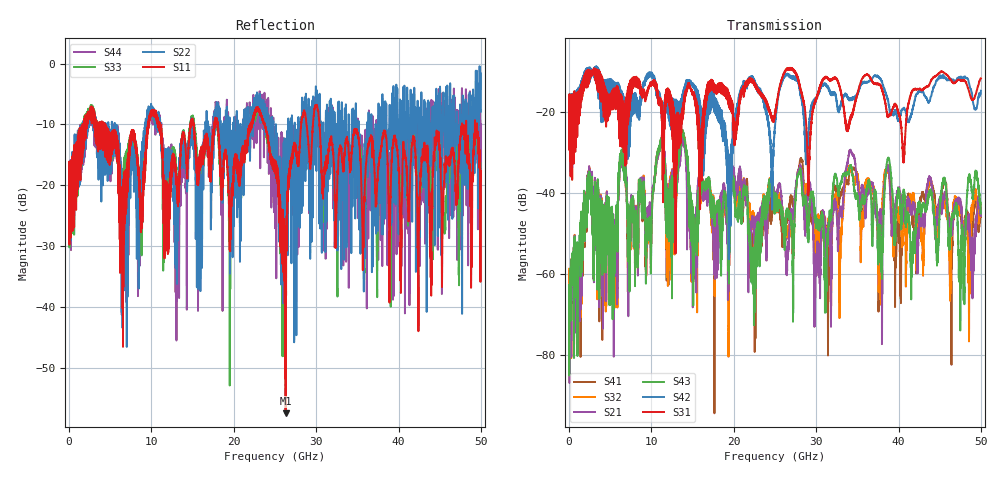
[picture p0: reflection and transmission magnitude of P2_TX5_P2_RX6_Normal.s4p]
!Keysight Technologies,N5225B,MY57041031,A.13.20.10
!Date: Friday, May 31, 2019 11:36:14
!Correction: S11(Full 4 Port(1,2,3,4))
!S12(Full 4 Port(1,2,3,4))
!S13(Full 4 Port(1,2,3,4))
!S14(Full 4 Port(1,2,3,4))
!S21(Full 4 Port(1,2,3,4))
!S22(Full 4 Port(1,2,3,4))
!S23(Full 4 Port(1,2,3,4))
!S24(Full 4 Port(1,2,3,4))
!S31(Full 4 Port(1,2,3,4))
!S32(Full 4 Port(1,2,3,4))
!S33(Full 4 Port(1,2,3,4))
!S34(Full 4 Port(1,2,3,4))
!S41(Full 4 Port(1,2,3,4))
!S42(Full 4 Port(1,2,3,4))
!S43(Full 4 Port(1,2,3,4))
!S44(Full 4 Port(1,2,3,4))
!S4P File: Measurements: <S11,S12,S13,S14>,
!<S21,S22,S23,S24>,
!<S31,S32,S33,S34>,
!<S41,S42,S43,S44>:
# Hz S  dB  R 50.0
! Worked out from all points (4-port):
!   5000 points, 10 MHz to 50 GHz, reference 50 ohm
!   strongest paths, dB at 10 MHz, 12.51 GHz, 25.01 GHz, 37.51 GHz, 50 GHz:
!     S31: -19.5, -17.7, -21.0, -13.1, -11.7
!     S42: -19.4, -16.8, -23.5, -11.2, -14.8
!     S43: -74.7, -40.7, -43.9, -52.8, -45.1
!     S21: -65.9, -37.4, -41.6, -51.0, -45.6
!     S32: -58.7, -37.5, -42.2, -56.1, -43.0
!     S41: -59.1, -39.3, -43.6, -54.7, -45.9
!   lowest |S11| = -57.5 dB at 26.29 GHz (marker M1), VSWR 1.00, Z = 50.1 - j0.0859 ohm
!   |S11| at or under -10 dB: 4.282 GHz to 9.568 GHz (5.286 GHz wide, 76.3 % of centre); 23.74 GHz to 28.18 GHz (4.441 GHz wide, 17.1 % of centre); 30.41 GHz to 47.7 GHz (17.29 GHz wide, 44.3 % of centre)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
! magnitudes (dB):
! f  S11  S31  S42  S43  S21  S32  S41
! 10 MHz  -19.9  -19.5  -19.4  -74.7  -65.9  -58.7  -59.1
! 6.39 GHz  -29.5  -25.3  -20.5  -30.7  -31.4  -31.2  -30.6
! 19.46 GHz  -25.2  -15.9  -32.3  -54.3  -50.7  -48.5  -57.9
! 26.29 GHz  -57.5  -9.7  -10.9  -46.8  -52.4  -49.4  -46.2
! 30.01 GHz  -6.8  -16.7  -17.0  -48.1  -56.0  -51.0  -53.5
! 34.19 GHz  -16.7  -21.7  -17.0  -33.3  -29.5  -33.7  -33.7
! 50 GHz  -19.2  -11.7  -14.8  -45.1  -45.6  -43.0  -45.9
